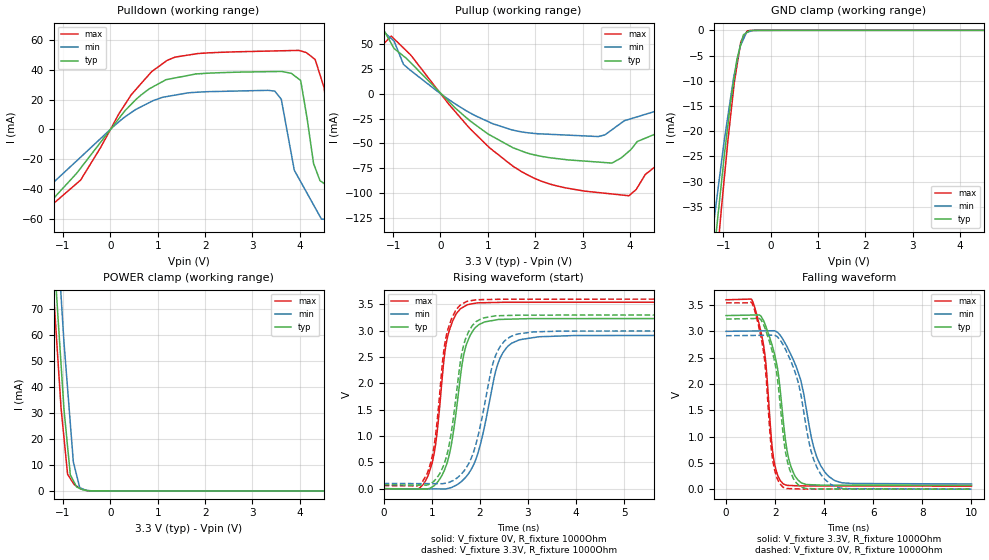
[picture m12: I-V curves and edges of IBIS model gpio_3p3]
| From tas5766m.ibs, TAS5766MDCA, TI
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|   gpio_3p3 Model
[Model]   gpio_3p3
Model_type   I/O
Polarity   Non-Inverting
Enable   Active-Low
Vinl = 0.99
Vinh = 2.31
Vmeas = 1.65
Vref = 0
Cref = 1pF
Rref = 1000000
|   typ   min   max
C_comp   1.371pF   1.337pF   1.391pF
[Voltage Range]   3.3   3   3.6
[Temperature Range]   27   105   -25
[Pullup Reference]   3.3   3   3.6
[Pulldown Reference]   -0   -0   -0
[Power Clamp Reference]   3.3   3   3.6
[GND Clamp Reference]   -0   -0   -0
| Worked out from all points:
|   slope of the pulldown table from 0 to 0.495 V, typ, clamps not added: 26.4 ohm
|   slope of the pullup table from 0 to 0.495 V, typ, clamps not added: 21.8 ohm
|   GND clamp passes 1 mA (typ) near -0.58 V on its own axis
|   POWER clamp passes 1 mA (typ) near -0.65 V on its own axis
|   falling waveform, V_fixture 3.3V, R_fixture 1000Ohm: 20-80 % time 568ps typ, 874ps min, 420ps max; typ from 3.3 V to 0.073 V
|   rising waveform, V_fixture 0V, R_fixture 1000Ohm: 20-80 % time 312ps typ, 435ps min, 261ps max; typ from 0 V to 3.23 V
|   rising waveform, V_fixture 3.3V, R_fixture 1000Ohm: 20-80 % time 309ps typ, 424ps min, 260ps max; typ from 0.073 V to 3.3 V
|   falling waveform, V_fixture 0V, R_fixture 1000Ohm: 20-80 % time 549ps typ, 830ps min, 410ps max; typ from 3.23 V to 0 V
[Pulldown]
|   Voltage   I(typ)   I(min)   I(max)
-3.3V     -1.19mA    -1.068mA   -1.279mA
-3.13V    -56.53mA   -55.88mA   -56.93mA
-2.96V    -65.45mA   -64.53mA   -66.01mA
-1.97V    -54.07mA   -42.32mA   -64.09mA
1.928V    37.49mA    25.13mA    51.11mA
3.471V    38.83mA    25.67mA    52.7mA
3.979V    33.81mA    -32.96mA   53.06mA
4.323V    -25.75mA   -52.64mA   46.99mA
4.833V    -60.8mA    -60.99mA   -27.81mA
5.401V    -62mA      -61.98mA   -63.02mA
6.4V      -64.12mA   -63.73mA   -65.05mA
6.6V      774.6mA    899.5mA    659.9mA
[GND Clamp]
|   Voltage   I(typ)   I(min)   I(max)
-3.3V     -527.4mA   -490.8mA   -553.6mA
-1.376V   -61.94mA   -52.32mA   -72.28mA
-1.178V   -42.72mA   -36.47mA   -50.11mA
-1.04V    -30.42mA   -26.36mA   -35.52mA
-903.2mV  -18.92mA   -17.07mA   -22mA
-845.4mV  -14.35mA   -13.44mA   -17.07mA
-765.8mV  -9.242mA   -8.708mA   -10.28mA
-711mV    -5.727mA   -6.208mA   -7.075mA
-628.5mV  -2.774mA   -2.891mA   -2.254mA
-576.6mV  -915.5uA   -1.812mA   -1.436mA
-491.1mV  -356.3uA   -386.3uA   -88.84uA
6.6V      0A         0A         0A
[Pullup]
|   Voltage   I(typ)   I(min)   I(max)
-3.3V     618.1uA    488.4uA    720.8uA
-3.13V    56.63mA    56.35mA    56.84mA
-2.96V    65.79mA    65.46mA    66.04mA
-1.376V   64.46mA    63.29mA    66.01mA
1.531V    -54.38mA   -36.65mA   -72.95mA
3.979V    -57.89mA   -25.79mA   -102.6mA
4.847V    -30.01mA   -10.87mA   -61.57mA
5.03V     -28.42mA   14.1mA     -54.71mA
5.619V    49.27mA    55.85mA    -10mA
6V        55.34mA    58.87mA    51.05mA
6.405V    57.16mA    62.08mA    47.59mA
6.6V      -529.1mA   -589.3mA   -458.7mA
[POWER Clamp]
|   Voltage   I(typ)   I(min)   I(max)
-3.3V     774.1mA    800.5mA    758.1mA
-1.376V   148.1mA    176.3mA    130.9mA
-1.178V   87.23mA    115.2mA    70.27mA
-1.04V    48.6mA     75.07mA    31.77mA
-979.8mV  31.54mA    57.35mA    20.58mA
-903.2mV  17.07mA    39.47mA    6.439mA
-845.4mV  6.18mA     26mA       4.775mA
-781.8mV  3.962mA    11.17mA    2.943mA
-711mV    1.491mA    5.978mA    1.811mA
-646.4mV  967.5uA    1.248mA    1.021mA
-576.6mV  401.3uA    714.5uA    527.2uA
6.6V      0A         0A         0A
[Ramp]
R_load = 1000
|   typ   min   max
dV/dt_r   1.93976/3.10881e-10   1.7498/4.33053e-10   2.12526/2.59591e-10
dV/dt_f   1.93625/5.6397e-10   1.74069/8.67744e-10   2.12484/4.1806e-10
[Falling Waveform]
V_fixture = 3.3V
V_fixture_min = 3V
V_fixture_max = 3.6V
R_fixture = 1000Ohm
C_fixture = 0F
|   Time   V(typ)   V(min)   V(max)
0s        3.3V       3V         3.6V
1.155ns   3.311V     3.007V     3.476V
1.585ns   3.14V      3.01V      2.555V
1.9ns     2.699V     3.012V     711.6mV
2.329ns   1.315V     2.838V     100.2mV
2.547ns   589.6mV    2.648V     71.12mV
2.829ns   236.9mV    2.361V     65.63mV
3.573ns   82.61mV    792.5mV    61.48mV
4.199ns   76.75mV    237.7mV    61.2mV
10ns      72.91mV    98.84mV    58.58mV
[Rising Waveform]
V_fixture = 0V
V_fixture_min = 0V
V_fixture_max = 0V
R_fixture = 1000Ohm
C_fixture = 0F
|   Time   V(typ)   V(min)   V(max)
0s        1.823nV    31.53nV    1.041nV
856.7ps   -8.873mV   -3.49mV    127.2mV
1.048ns   57.43mV    -4.269mV   658.8mV
1.195ns   223.3mV    -4.866mV   1.866V
1.359ns   622mV      10.05mV    2.986V
1.738ns   2.779V     253.7mV    3.491V
2.011ns   3.128V     839.6mV    3.529V
2.396ns   3.213V     2.424V     3.537V
2.806ns   3.223V     2.82V      3.539V
10ns      3.233V     2.916V     3.542V
[Rising Waveform]
V_fixture = 3.3V
V_fixture_min = 3V
V_fixture_max = 3.6V
R_fixture = 1000Ohm
C_fixture = 0F
|   Time   V(typ)   V(min)   V(max)
0s        72.78mV    98.58mV    58.46mV
800.2ps   68.19mV    95.96mV    122.7mV
1.034ns   132.8mV    95.2mV     726.9mV
1.169ns   290.3mV    94.76mV    1.841V
1.343ns   746.2mV    116mV      3.047V
1.715ns   2.872V     396.2mV    3.549V
1.925ns   3.174V     868mV      3.586V
2.331ns   3.282V     2.536V     3.594V
2.734ns   3.292V     2.922V     3.597V
10ns      3.3V       3V         3.6V
[Falling Waveform]
|Gnd
V_fixture = 0V
V_fixture_min = 0V
V_fixture_max = 0V
R_fixture = 1000Ohm
C_fixture = 0F
|   Time   V(typ)   V(min)   V(max)
0s        3.233V     2.917V     3.542V
1.13ns    3.244V     2.922V     3.452V
1.559ns   3.093V     2.925V     2.503V
1.875ns   2.629V     2.926V     645.9mV
2.312ns   1.109V     2.754V     40.77mV
2.501ns   522.7mV    2.579V     11.91mV
2.876ns   111.9mV    2.129V     5.514mV
3.564ns   7.747mV    570.9mV    2.707mV
4.284ns   3.931mV    86.11mV    2.418mV
10ns      126.1uV    245.5uV    120.5uV
